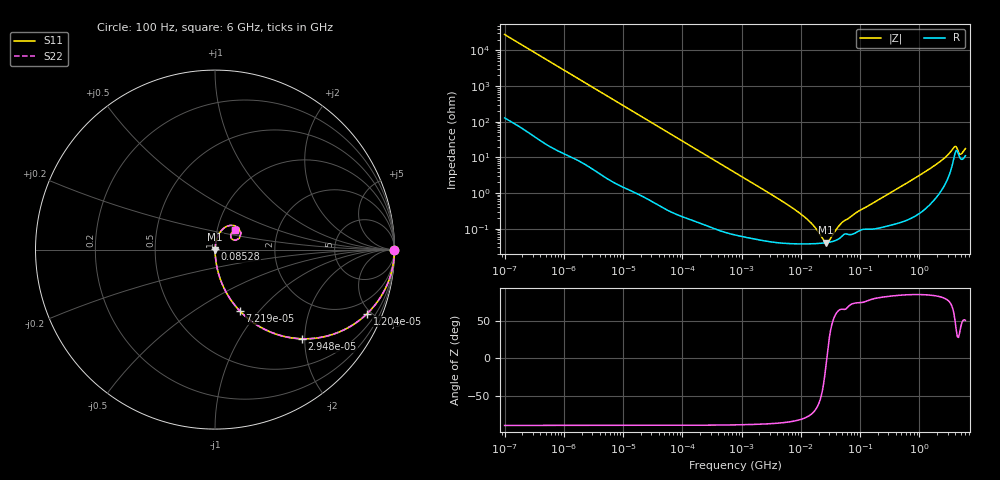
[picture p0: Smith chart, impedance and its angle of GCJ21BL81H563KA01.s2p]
!Murata Part Number: GCJ21BL81H563KA01
!These Parameters are Measured in Series Mode Connection
!Data Generated on Mar 13, 2026
!  o--ll--o
!Port1  Port2
!  o------o
!Operation Temp=25[degC], DC Bias Voltage=0[V]
!Freq. Start=100[Hz] Stop=6[GHz] 401[Steps]
# Hz S RI R 50
!Freq.(Hz) S11(Real) S11(Imag) S21(Real) S21(Imag) S12(Real) S12(Imag) S22(Real) S22(Imag)
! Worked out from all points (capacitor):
!   401 points, 100 Hz to 6 GHz, reference 50 ohm
!   read as one part in series: C = 56.5 nF near 109 Hz
!   lowest |Z| = 40.7 mohm at 26.62 MHz (marker M1)
!   series resonance near 27.44 MHz, so ESL is about 600 pH
!   S11 on the Smith chart (normalised r, x): 100 Hz: open; 12.04 kHz: 1.03, -4.74; 29.48 kHz: 1.01, -1.94; 72.19 kHz: 1.01, -0.80; 85.28 MHz: 1.00, +0.01; 6 GHz: 1.22, +0.27
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100  1 -0.00355  2.88e-05 0.00355  2.88e-05 0.00355  1 -0.00355
2008  0.9947 -0.0704  0.00534 0.0704  0.00534 0.0704  0.9947 -0.0704
5882  0.9582 -0.1977  0.0418 0.1977  0.0418 0.1977  0.9582 -0.1977
12041  0.8475 -0.3569  0.1525 0.3569  0.1525 0.3569  0.8475 -0.3569
29482  0.4854 -0.4967  0.5146 0.4967  0.5146 0.4967  0.4854 -0.4967
40335  0.3365 -0.4694  0.6635 0.4694  0.6635 0.4694  0.3365 -0.4694
72189  0.1383 -0.3418  0.8617 0.3418  0.8617 0.3418  0.1383 -0.3418
211427  0.0196 -0.1336  0.9804 0.1336  0.9804 0.1336  0.0196 -0.1336
774597  0.00206 -0.0373  0.9979 0.0373  0.9979 0.0373  0.00206 -0.0373
6644369  0.000395 -0.00416  0.9996 0.00416  0.9996 0.00416  0.000395 -0.00416
1.555665e7  0.000377 -0.00128  0.9996 0.00128  0.9996 0.00128  0.000377 -0.00128
2.434276e7  0.000394 -0.000258  0.9996 0.000258  0.9996 0.000258  0.000394 -0.000258
2.662322e7  0.000401 -6.44e-05  0.9996 6.44e-05  0.9996 6.44e-05  0.000401 -6.44e-05
3.045065e7  0.000416 0.000226  0.9996 -0.000226  0.9996 -0.000226  0.000416 0.000226
4.764863e7  0.000576 0.00126  0.9994 -0.00126  0.9994 -0.00126  0.000576 0.00126
8.527865e7  0.000779 0.00267  0.9992 -0.00267  0.9992 -0.00267  0.000779 0.00267
3.124326e8  0.00131 0.00965  0.9987 -0.00965  0.9987 -0.00965  0.00131 0.00965
1.791126e9  0.00962 0.057  0.9904 -0.057  0.9904 -0.057  0.00962 0.057
2.931063e9  0.0328 0.1029  0.9672 -0.1029  0.9672 -0.1029  0.0328 0.1029
3.8344e9  0.1064 0.1343  0.8936 -0.1343  0.8936 -0.1343  0.1064 0.1343
5.016141e9  0.0881 0.0684  0.9119 -0.0684  0.9119 -0.0684  0.0881 0.0684
6e9  0.1134 0.1084  0.8866 -0.1084  0.8866 -0.1084  0.1134 0.1084
